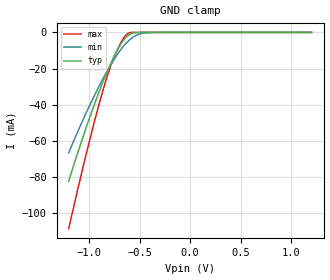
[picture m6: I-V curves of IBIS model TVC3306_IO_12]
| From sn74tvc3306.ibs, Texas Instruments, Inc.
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[Model]   TVC3306_IO_12
Model_type  Terminator
| variable   typ   min   max
C_comp   2.91pF   2.56pF   3.28pF
| C_tri-state   2.91pF   2.56pF   3.28pF
[Temperature Range]   40   100   -40
| Ambient temperature   25   85   -40
[Voltage range]   1.2   1.2   1.2
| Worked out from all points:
|   GND clamp passes 1 mA (typ) near -0.59 V on its own axis
[GND Clamp]
| TVC3306_IO_12
|   Voltage   I(typ)   I(min)   I(max)
-1.2V     -82.18mA   -66.55mA   -108.4mA
-1V       -48.23mA   -41.19mA   -61.2mA
-915mV    -35.1mA    -31.42mA   -42.81mA
-840mV    -24.41mA   -23.43mA   -27.99mA
-785mV    -17.27mA   -18.04mA   -18.52mA
-730mV    -10.92mA   -13.12mA   -10.85mA
-670mV    -5.288mA   -8.435mA   -4.262mA
-620mV    -2.059mA   -5.247mA   -792.2uA
-575mV    -509.5uA   -3.113mA   -31.16uA
-520mV    -89.48uA   -1.362mA   -3.481uA
-405mV    -2.569uA   -120.3uA   -35.6nA
1.2V      17.63pA    2.878nA    5.13pA
